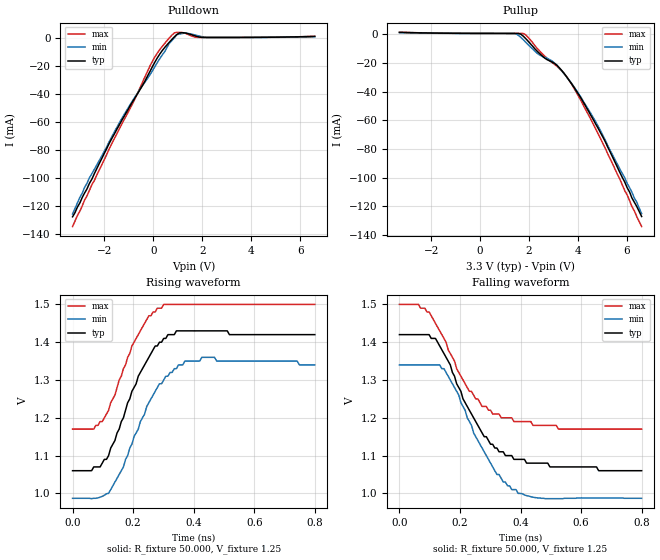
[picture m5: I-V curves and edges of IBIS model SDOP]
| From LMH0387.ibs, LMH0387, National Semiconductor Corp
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|   Model SDOP
[Model]  SDOP
Model_type Output
Polarity   Non-Inverting
Vmeas =  1.2V
Rref =   50.0000
Vref =   1.20V
C_comp   542.2fF   513.0fF   577.4fF
[Temperature Range]   34.0000   94.0000   -31.0000
[Voltage Range]   3.3000V   3.1350V   3.4650V
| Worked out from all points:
|   slope of the pulldown table from 0 to 0.495 V, typ, clamps not added: 37.7 ohm
|   slope of the pullup table from 0 to 0.495 V, typ, clamps not added: 38.1 kohm
|   rising waveform, R_fixture 50.000, V_fixture 1.25: 20-80 % time 109ps typ, 113ps min, 102ps max; typ from 1.06 V to 1.42 V
|   falling waveform, R_fixture 50.000, V_fixture 1.25: 20-80 % time 137ps typ, 127ps min, 139ps max; typ from 1.42 V to 1.06 V
[Pulldown]
|Voltage   I(typ)   I(min)   I(max)
-3.3V     -128mA     -126mA     -135mA
-2.61V    -104mA     -100mA     -109mA
-1.32V    -59.9mA    -58.5mA    -62.7mA
-825mV    -44.9mA    -44.2mA    -46.2mA
-33mV     -20.3mA    -23.3mA    -16.4mA
363mV     -8.95mA    -12.1mA    -5.95mA
660mV     -2.8mA     -3.59mA    273uA
858mV     928uA      193uA      3.75mA
1.06V     3.72mA     2.99mA     4.23mA
1.35V     3.58mA     3.59mA     3.19mA
2.05V     540uA      862uA      551uA
6.6V      1.31mA     993uA      1.3mA
[Pullup]
|Voltage   I(typ)   I(min)   I(max)
-3.3V     1.31mA     993uA      1.3mA
1.35V     516uA      476uA      550uA
1.65V     98.8uA     -2.04mA    546uA
1.85V     -2.87mA    -5.37mA    -326uA
2.34V     -12mA      -13.4mA    -10.1mA
2.64V     -16.7mA    -16.2mA    -15.3mA
3.14V     -21.7mA    -21.7mA    -22.4mA
3.53V     -29.6mA    -29.7mA    -29.5mA
3.93V     -39.5mA    -39mA      -40.5mA
4.92V     -68.7mA    -67.3mA    -72.8mA
5.91V     -103mA     -100mA     -109mA
6.6V      -127mA     -125mA     -134mA
[Ramp]
|variable   typ   min   max
dV/dt_r   215.21m/105.7p   214.09m/131.1p   200.36m/99.93p
dV/dt_f   215.31m/126.8p   213.97m/129.6p   200.43m/123.8p
R_load  = 50
[Rising Waveform]
R_fixture = 50.000
V_fixture = 1.25
V_fixture_min = 1.125
V_fixture_max = 1.375
|  time   V(typ)   V(min)   V(max)
0s        1.06V      987mV      1.17V
70ps      1.07V      987mV      1.17V
119ps     1.1V       1V         1.22V
168ps     1.2V       1.07V      1.33V
217ps     1.31V      1.17V      1.42V
252ps     1.36V      1.24V      1.47V
315ps     1.42V      1.31V      1.5V
371ps     1.43V      1.35V      1.5V
427ps     1.43V      1.36V      1.5V
800ps     1.42V      1.34V      1.5V
[Falling Waveform]
R_fixture = 50.000
V_fixture = 1.25
V_fixture_min = 1.125
V_fixture_max = 1.375
|  time   V(typ)   V(min)   V(max)
0s        1.42V      1.34V      1.5V
84ps      1.42V      1.34V      1.49V
119ps     1.41V      1.34V      1.45V
147ps     1.37V      1.33V      1.41V
231ps     1.22V      1.19V      1.27V
280ps     1.15V      1.11V      1.23V
322ps     1.12V      1.05V      1.21V
392ps     1.09V      1V         1.19V
525ps     1.07V      986mV      1.17V
800ps     1.06V      987mV      1.17V
